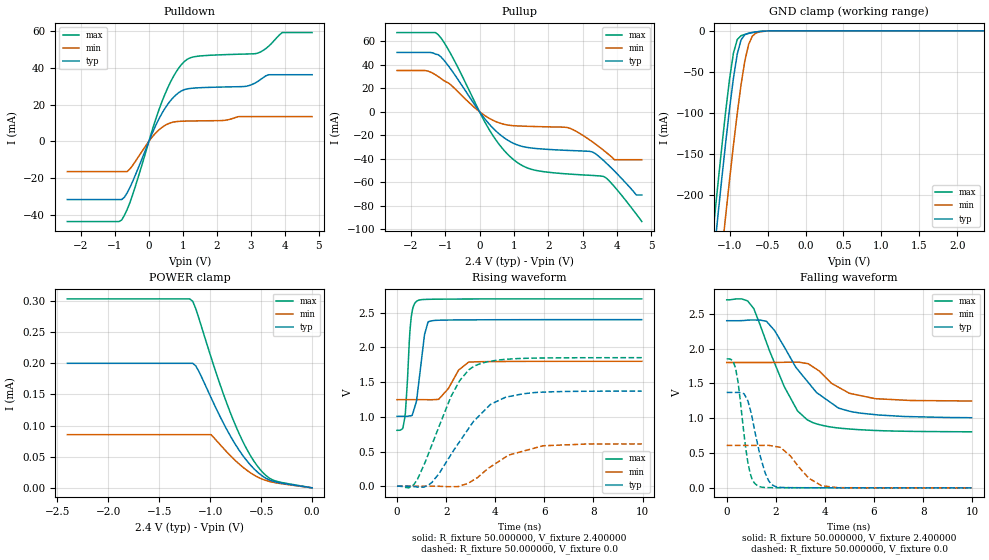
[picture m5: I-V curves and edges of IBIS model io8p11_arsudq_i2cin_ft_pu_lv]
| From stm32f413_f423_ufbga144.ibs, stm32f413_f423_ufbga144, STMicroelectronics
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|   Model io8p11_arsudq_i2cin_ft_pu_lv
[Model]  io8p11_arsudq_i2cin_ft_pu_lv
Model_type I/O
Polarity   Non-Inverting
Enable   Active-Low
Vinl =   0.720000V
Vinh =   1.680000V
Vmeas =  1.200000V
Cref =   30.000000pF
Rref =   100.000000M
Vref =   0.0V
C_comp   2.230300pF   2.174000pF   2.332300pF
[Temperature Range]   25.000000   0.125000k   -40.000000
[Pullup Reference]   2.400000V   1.800000V   2.700000V
[Pulldown Reference]   0.0V   0.0V   0.0V
[POWER Clamp Reference]   2.400000V   1.800000V   2.700000V
[GND Clamp Reference]   0.0V   0.0V   0.0V
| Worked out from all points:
|   slope of the pulldown table from 0 to 0.36 V, typ, clamps not added: 25 ohm
|   slope of the pullup table from 0 to 0.36 V, typ, clamps not added: 27.7 ohm
|   GND clamp passes 1 mA (typ) near -0.62 V on its own axis
|   rising waveform, R_fixture 50.000000, V_fixture 2.400000: 20-80 % time 284ps typ, 603ps min, 184ps max; typ from 1.01 V to 2.4 V
|   rising waveform, R_fixture 50.000000, V_fixture 0.0: 20-80 % time 1.7ns typ, 1.69ns min, 1.32ns max; typ from 0.001 V to 1.37 V
|   falling waveform, R_fixture 50.000000, V_fixture 2.400000: 20-80 % time 1.81ns typ, 1.29ns min, 1.38ns max; typ from 2.4 V to 1.01 V
|   falling waveform, R_fixture 50.000000, V_fixture 0.0: 20-80 % time 536ps typ, 925ps min, 385ps max; typ from 1.37 V to 0.001 V
[Pulldown]
|Voltage   I(typ)   I(min)   I(max)
-2.4V     -31.73mA   -16.51mA   -43.74mA
-800mV    -31.73mA   -16.51mA   -42.87mA
-480mV    -21.98mA   -13.17mA   -29.21mA
80mV      3.63mA     1.966mA    5.014mA
480mV     18.16mA    8.738mA    26.02mA
800mV     25.38mA    10.72mA    37.77mA
1.12V     28.53mA    11.02mA    44.6mA
2.8V      29.84mA    13.46mA    47.53mA
3.2V      32.6mA     13.46mA    48.03mA
3.52V     36.28mA    13.46mA    51.75mA
3.92V     36.28mA    13.46mA    59.24mA
4.8V      36.28mA    13.46mA    59.24mA
[Pullup]
|Voltage   I(typ)   I(min)   I(max)
-2.4V     50.44mA    35.08mA    67.32mA
-1.52V    50.44mA    34.74mA    67.32mA
-1.2V     48.5mA     29.88mA    65.48mA
320mV     -11.75mA   -6.207mA   -17.08mA
1.04V     -27.53mA   -11.97mA   -41.91mA
1.6V      -31.13mA   -12.57mA   -49.63mA
2.56V     -32.88mA   -13.48mA   -52.9mA
3.28V     -34.18mA   -25.52mA   -54.17mA
3.6V      -41.3mA    -32.61mA   -54.97mA
3.92V     -50.32mA   -40.8mA    -63.62mA
4.56V     -70.8mA    -40.8mA    -87.07mA
4.72V     -70.8mA    -40.8mA    -93.4mA
[GND_clamp]
|Voltage   I(typ)   I(min)   I(max)
-2.4V     -1.424A    -1.508A    -1.393A
-1.25V    -311.2mA   -401.9mA   -273.3mA
-1.2V     -265.4mA   -356.1mA   -227.2mA
-1.15V    -220.4mA   -310.8mA   -181.9mA
-1.1V     -176.3mA   -266.2mA   -137.9mA
-1.05V    -133.8mA   -222.5mA   -95.87mA
-950mV    -57.3mA    -138.9mA   -26.98mA
-900mV    -28.27mA   -100.4mA   -10.59mA
-850mV    -11.01mA   -65.54mA   -5.958mA
-750mV    -2.834mA   -16.5mA    -3.178mA
-600mV    -750uA     -1.164mA   -738.3uA
2.35V     0A         0A         0A
[POWER_clamp]
|Voltage   I(typ)   I(min)   I(max)
-2.4V     200uA      85.39uA    303.5uA
-1.2V     200uA      85.39uA    303.5uA
-1.17V    200uA      85.39uA    299.5uA
-1.14V    195.7uA    85.39uA    287.5uA
-990mV    144.6uA    85.39uA    209.3uA
-870mV    104.1uA    63.61uA    150.8uA
-780mV    77.28uA    48.2uA     111.8uA
-660mV    47.71uA    30.75uA    68.21uA
-570mV    30.64uA    20.61uA    42.79uA
-480mV    18.19uA    13.44uA    24.07uA
-390mV    10.91uA    9.231uA    13.01uA
0V        0A         0A         0A
[Ramp]
| variable   typ   min   max
dV/dt_r  0.82159/1.69576n   0.36425/1.67900n   1.11077/1.31603n
dV/dt_f  0.83190/1.80511n   0.33228/1.29979n   1.13489/1.38036n
R_load = 50.000000
[Rising Waveform]
R_fixture= 50.000000
V_fixture= 2.400000
V_fixture_min= 1.800000
V_fixture_max= 2.700000
|time   V(typ)   V(min)   V(max)
0s        1.007V     1.247V     805.7mV
240.2ps   1.007V     1.247V     838.9mV
320.3ps   1.007V     1.247V     995.1mV
580.6ps   1.017V     1.247V     2.443V
820.8ps   1.305V     1.247V     2.67V
1.121ns   2.187V     1.247V     2.691V
1.281ns   2.37V      1.246V     2.693V
1.702ns   2.392V     1.254V     2.695V
2.923ns   2.397V     1.788V     2.698V
9.97ns    2.4V       1.8V       2.699V
[Rising Waveform]
R_fixture= 50.000000
V_fixture= 0.0
V_fixture_min= 0.0
V_fixture_max= 0.0
|time   V(typ)   V(min)   V(max)
0s        1.05mV     906.2uV    1.445mV
680.7ps   -4.598mV   892.7uV    23.35mV
1.421ns   55.01mV    970.5uV    597.5mV
2.202ns   458.6mV    -6.025mV   1.295V
2.563ns   649.7mV    4.019mV    1.526V
3.143ns   943.3mV    95.69mV    1.73V
3.804ns   1.179V     278.5mV    1.8V
4.424ns   1.283V     421.6mV    1.828V
5.946ns   1.356V     582.9mV    1.848V
9.97ns    1.371V     610.1mV    1.852V
[Falling Waveform]
R_fixture= 50.000000
V_fixture= 2.400000
V_fixture_min= 1.800000
V_fixture_max= 2.700000
|time   V(typ)   V(min)   V(max)
0s        2.4V       1.8V       2.699V
620.6ps   2.401V     1.8V       2.711V
1.101ns   2.41V      1.8V       2.574V
1.622ns   2.39V      1.8V       2.085V
2.342ns   2.025V     1.803V     1.454V
2.883ns   1.702V     1.805V     1.105V
3.283ns   1.53V      1.785V     977.3mV
4.545ns   1.148V     1.447V     860.2mV
5.125ns   1.091V     1.349V     842.4mV
9.97ns    1.007V     1.247V     805.7mV
[Falling Waveform]
R_fixture= 50.000000
V_fixture= 0.0
V_fixture_min= 0.0
V_fixture_max= 0.0
|time   V(typ)   V(min)   V(max)
0s        1.371V     610.1mV    1.852V
360.4ps   1.371V     610.2mV    1.716V
460.5ps   1.37V      610.1mV    1.52V
720.7ps   1.343V     610.1mV    721.1mV
961ps     1.12V      609.9mV    201mV
1.281ns   589.4mV    609.8mV    27.6mV
1.702ns   107mV      610.8mV    4.384mV
2.062ns   13.46mV    590.3mV    3.236mV
3.864ns   1.992mV    31.45mV    2.235mV
9.97ns    1.05mV     906.2uV    1.445mV
